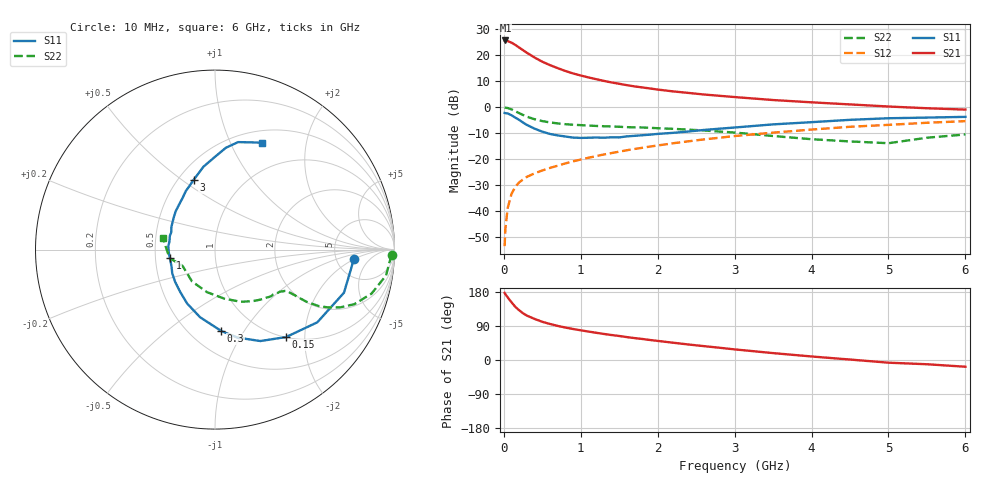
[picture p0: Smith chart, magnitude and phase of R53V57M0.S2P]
! SIEMENS Small Signal Semiconductors
! BFR183
! Si NPN RF Bipolar Junction Transistor in SOT23
! VCE = 3.5 V  IC = 7 mA
! Common Emitter S-Parameters:  May  1996
# GHz  S  MA  R  50
!  f  S11  S21  S12  S22
! GHz  MAG  ANG  MAG  ANG  MAG  ANG  MAG  ANG
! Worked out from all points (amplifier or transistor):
!   36 points, 10 MHz to 6 GHz, reference 50 ohm
!   highest |S21| = 25.7 dB at 20 MHz (marker M1)
!   |S21| within 3 dB of that: start of sweep to 212.8 MHz
!   unconditionally stable (mu >= 1): 881.7 MHz to 2.558 GHz
!   at 250 MHz: K = 0.51, MSG = 24.9 dB, |S12| = -27.8 dB
!   at 1.4 GHz: K = 1.06, MAG = 12.1 dB, |S12| = -17.7 dB
!   at 6 GHz: K = 0.88, MSG = 2.2 dB, |S12| = -5.4 dB
!   lowest NFmin = 1.25 dB at 450 MHz
!   S11 on the Smith chart (normalised r, x): 10 MHz: 7.38, -1.89; 150 MHz: 1.01, -1.62; 300 MHz: 0.70, -0.80; 1 GHz: 0.60, -0.06; 3 GHz: 0.60, +0.55; 6 GHz: 0.64, +1.33
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0.01  0.7746 -3.8  19.19 177.0  0.0021 85.5  0.9843 -1.7
0.02  0.7666 -7.5  19.31 173.7  0.0045 85.2  0.977 -3.5
0.05  0.7577 -18.5  18.77 165.3  0.0114 80.1  0.9638 -8.6
0.1  0.6994 -35.4  17.51 152.3  0.0214 73.6  0.906 -15.7
0.15  0.6278 -50.9  15.8 140.1  0.0293 68.4  0.8337 -21.4
0.2  0.5688 -63.6  14.09 131.1  0.0357 64.0  0.7676 -24.8
0.25  0.5058 -75.7  12.53 123.2  0.0406 61.3  0.7072 -27.1
0.3  0.4548 -85.6  11.17 117.1  0.0455 60.5  0.6566 -28.6
0.4  0.3857 -102.5  9.054 108.4  0.0532 59.1  0.5863 -29.7
0.5  0.3379 -117.4  7.514 100.8  0.0604 59.7  0.54 -29.8
0.6  0.3049 -129.6  6.465 95.0  0.0676 59.9  0.5088 -29.8
0.7  0.2859 -140.9  5.652 90.0  0.0746 60.8  0.4869 -29.9
0.8  0.2724 -151.0  4.987 85.6  0.0826 61.1  0.4704 -30.0
1  0.2559 -169.1  4.076 78.3  0.0982 61.8  0.451 -30.7
1.1  0.2579 -176.7  3.746 75.1  0.106 62.0  0.4431 -31.7
1.6  0.2741 152.3  2.655 60.4  0.1481 61.3  0.4126 -36.8
2.2  0.3205 128.7  2.015 45.6  0.2018 57.8  0.383 -46.0
3  0.406 107.1  1.568 28.0  0.278 50.3  0.3247 -63.6
3.5  0.4665 97.9  1.374 18.2  0.3232 44.5  0.2786 -79.1
4.5  0.5706 83.9  1.131 1.2  0.4193 32.5  0.2189 -125.8
5.5  0.6304 71.4  0.954 -11.2  0.5011 20.3  0.2581 -169.6
6  0.6513 66.1  0.899 -17.8  0.5388 12.4  0.2984 167.2
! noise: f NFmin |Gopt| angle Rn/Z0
0.45  1.25  0.18  42  0.22
0.9  1.3  0.22  110  0.2
1.8  2  0.33  180  0.14
